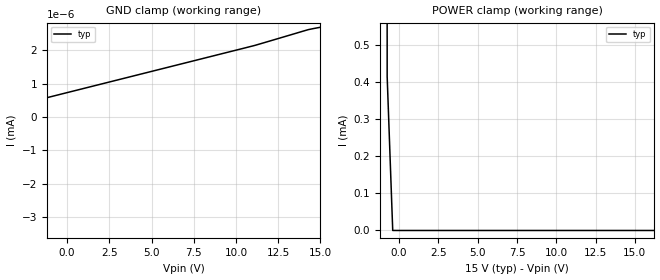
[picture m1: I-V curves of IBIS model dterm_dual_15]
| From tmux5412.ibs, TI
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| dterm_dual_15
[Model]   dterm_dual_15
Model_type   Terminator
|   typ   min   max
C_comp   1.008417e-11   NA   NA
[Voltage Range]   15   NA   NA
[Temperature Range]   27   NA   NA
[Power Clamp Reference]   15   NA   NA
[GND Clamp Reference]   0   NA   NA
[GND Clamp]
|   Voltage   I(typ)   I(min)   I(max)
-20V      -2.839A    NA         NA
-15.4V    -221.5nA   NA         NA
-15.05V   -1.213nA   NA         NA
-14.34V   -1.14nA    NA         NA
-11.16V   -686pA     NA         NA
11.11V    2.144nA    NA         NA
14.29V    2.618nA    NA         NA
15V       2.688nA    NA         NA
[POWER Clamp]
|   Voltage   I(typ)   I(min)   I(max)
-5V       2.61A      NA         NA
-1.111V   49.05mA    NA         NA
-757.6mV  413.6uA    NA         NA
-404mV    43.94nA    NA         NA
30V       -1.209nA   NA         NA
